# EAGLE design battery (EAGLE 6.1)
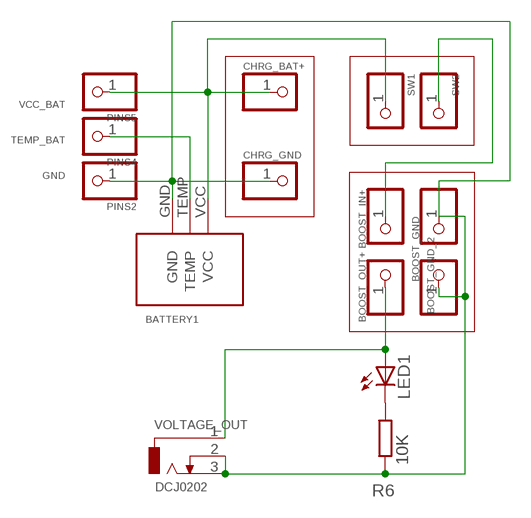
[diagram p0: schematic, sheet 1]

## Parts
BATTERY1  BAT-CASIO-NP40BATTERY  [BAT-CASIO-NP40]
BOOST_GND  PINHD-1X1CB  [1X01-CLEANBIG]
BOOST_GND_2  PINHD-1X1CB  [1X01-CLEANBIG]
BOOST_IN+  PINHD-1X1CB  [1X01-CLEANBIG]
BOOST_OUT+  PINHD-1X1CB  [1X01-CLEANBIG]
CHRG_BAT+  PINHD-1X1CB  [1X01-CLEANBIG]
CHRG_GND  PINHD-1X1CB  [1X01-CLEANBIG]
LED1  LED3MM  [LED3MM]
PINS2  PINHD-1X1CB  [1X01-CLEANBIG]
PINS4  PINHD-1X1CB  [1X01-CLEANBIG]
PINS5  PINHD-1X1CB  [1X01-CLEANBIG]
R6  10K  R-EU_0204/7  [0204/7]
SW1  PINHD-1X1CB  [1X01-CLEANBIG]
SW2  PINHD-1X1CB  [1X01-CLEANBIG]
VOLTAGE_OUT  DCJ0202  [DCJ0202]

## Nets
GND: BATTERY1.GND BOOST_GND.1 BOOST_GND_2.1 CHRG_GND.1 PINS2.1 R6.1 VOLTAGE_OUT.2 VOLTAGE_OUT.3
N$3: BOOST_IN+.1 SW2.1
N$7: LED1.K(C) R6.2
TEMP_BAT: BATTERY1.TEMP PINS4.1
VCC_BAT: BATTERY1.VCC CHRG_BAT+.1 PINS5.1 SW1.1
VCC_OUT: BOOST_OUT+.1 LED1.A VOLTAGE_OUT.1

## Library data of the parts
BATTERY1 = uradmonitor:BAT-CASIO-NP40: Li-ion 3.7V 1500mAh battery , compatible with Casio-NP-40
BOOST_GND BOOST_GND_2 BOOST_IN+ BOOST_OUT+ CHRG_BAT+ CHRG_GND PINS2 PINS4 PINS5 SW1 SW2 = adafruit:PINHD-1X1: Pin header 1x1 for 0.1" spacing
LED1 = adafruit:LED: LED
R6 = rcl:R-EU_: RESISTOR, European symbol
VOLTAGE_OUT = con-jack:DCJ0202: DC POWER JACK Source: DCJ0202.pdf; OC_FARNELL: unknown; OC_NEWARK: unknown

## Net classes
1 power: width 0.254 mm

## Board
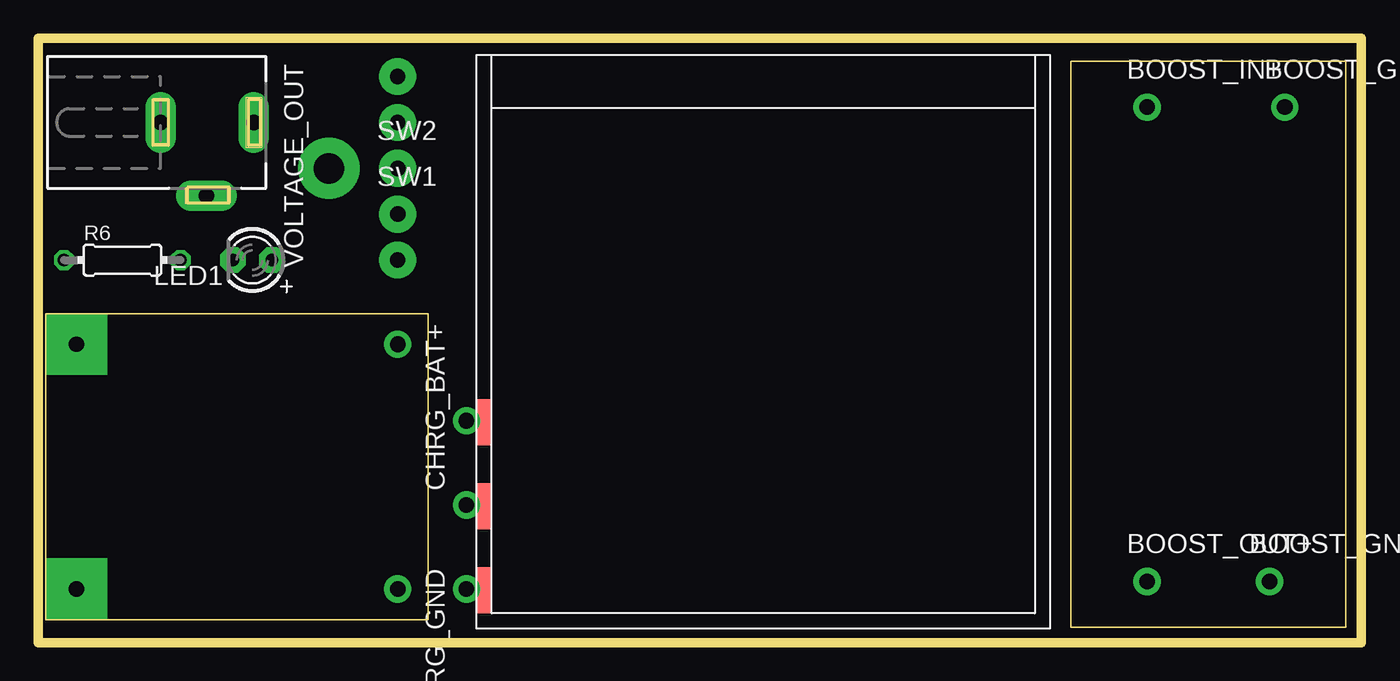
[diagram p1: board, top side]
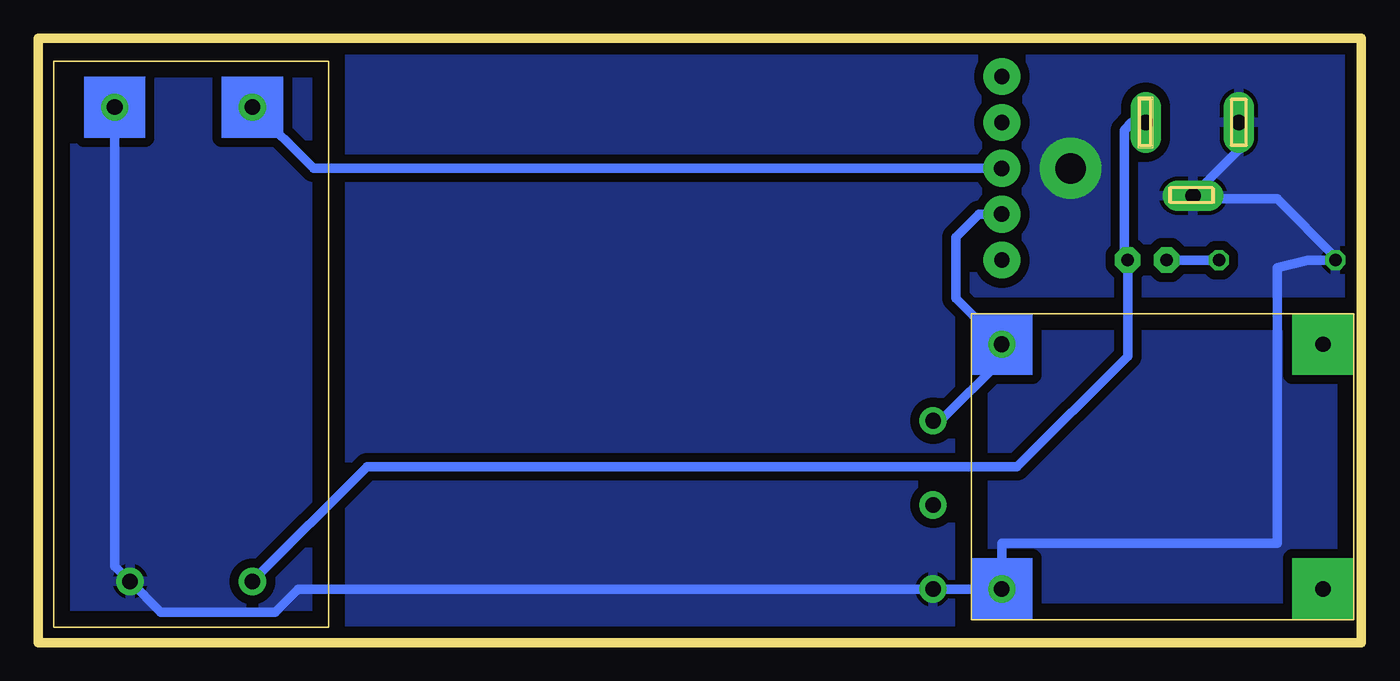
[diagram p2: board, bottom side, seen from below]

Size 86.5 x 39.5 mm. Coordinates in mm from the lower left corner, seen from the top.
Outline: 0.5,1.5 25.5,1.5 25.5,21.5 0.5,21.5 0.5,1.5
Outline: 67.5,38 85.5,38 85.5,1 67.5,1 67.5,38
Outline: 0,39.5 86.5,39.5 86.5,0 0,0 0,39.5
Copper layers (1*16): Top 0.035mm / dielectric 1.5mm / Bottom 0.035mm
Design rules: minimum track width 10mil, minimum drill 24mil, track to track 8mil, track to pad 8mil, pad to pad 8mil, via to via 8mil, smd to smd 8mil, copper to edge 40mil, drill to drill 8mil, minimum pad ring 10mil, minimum via ring 8mil, stop-mask expansion 4mil, vias tented up to drill 0mil, thermal gap 10mil
Milling: 16 lines

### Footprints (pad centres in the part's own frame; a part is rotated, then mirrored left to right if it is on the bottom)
BAT-CASIO-NP40 = smd 3 x 1: GND 34.59,-36.85; TEMP 29.09,-36.85; VCC 23.59,-36.85
1X01-CLEANBIG = drill 1.016 pad 1.778: 1 0,0
LED3MM = drill 0.813 pad 1.676 octagon: A -1.27,0; K 1.27,0
0204/7 = drill 0.813 octagon: 1 -3.81,0; 2 3.81,0
DCJ0202 = drill 1 pad 2 long: 1 0,3.1; 2 4.8,0; 3 0,-3

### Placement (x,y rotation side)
BATTERY1  66,38 270 top
BOOST_GND  81.5,35 0 top
BOOST_GND_2  80.5,4 0 top
BOOST_IN+  72.5,35 0 top
BOOST_OUT+  72.5,4 0 top
CHRG_BAT+  23.5,19.5 270 top
CHRG_GND  23.5,3.5 270 top
LED1  14,25 180 top
PINS2  28,3.5 180 top
PINS4  28,9 180 top
PINS5  28,14.5 180 top
R6  5.5,25 0 top
SW1  23.5,28 0 top
SW2  23.5,31 0 top
VOLTAGE_OUT  11,34 270 top

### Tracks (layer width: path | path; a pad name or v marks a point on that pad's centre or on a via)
GND  (via drill 2 pad 4)
  Top 0.61: PINS2.1 29.15,3.5 BATTERY1.GND
  Bottom 0.61: BOOST_GND.1 81.5,5 BOOST_GND_2.1 78.5,2 71,2 69.5,3.5 PINS2.1 CHRG_GND.1 23.5,6.5 5.5,6.5 5.5,20 5.5,24.5 3.5,25 R6.1 1.69,25.19 5.5,29 10.8,29 VOLTAGE_OUT.2 8,32.2 VOLTAGE_OUT.3
  other vias: 19,31
  pour Bottom (isolate 0.6): 0,39.5 86.5,39.5 86.5,0 0,0
N$1  (via drill 1 pad 4)
  other vias: 2.5,19.5
N$2  (via drill 1 pad 4)
  other vias: 2.5,3.5
N$3
  Bottom 0.61: SW2.1 68.5,31 BOOST_IN+.1
N$4  (via drill 1 pad 2.4)
  other vias: 23.5,28
N$5  (via drill 1 pad 2.4)
  other vias: 23.5,31
N$6  (via drill 1 pad 2.4)
  other vias: 23.5,34
N$7
  Bottom 0.61: LED1.K R6.2
N$8  (via drill 1 pad 2.4)
  other vias: 23.5,37
N$43452  (via drill 1 pad 2.4)
  other vias: 23.5,25
TEMP_BAT
  Top 0.61: PINS4.1 29.15,9 BATTERY1.TEMP
VCC_BAT
  Top 0.305: 29.14,15.55 BATTERY1.VCC 29.07,14.17 28.96,14.06 29.27,13.74
  Top 0.61: PINS5.1 29.15,14.5 BATTERY1.VCC
  Bottom 0.61: PINS5.1 27.5,14.5 23.5,18.5 CHRG_BAT+.1 26.5,22.5 26.5,26.5 25,28 SW1.1
VCC_OUT
  Bottom 0.61: VOLTAGE_OUT.1 15,34 15.5,33.5 15.5,25.23 LED1.A 15.27,18.73 22.5,11.5 65,11.5 BOOST_OUT+.1
(copper drawn outside any net)
  shapes: Bottom area x4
